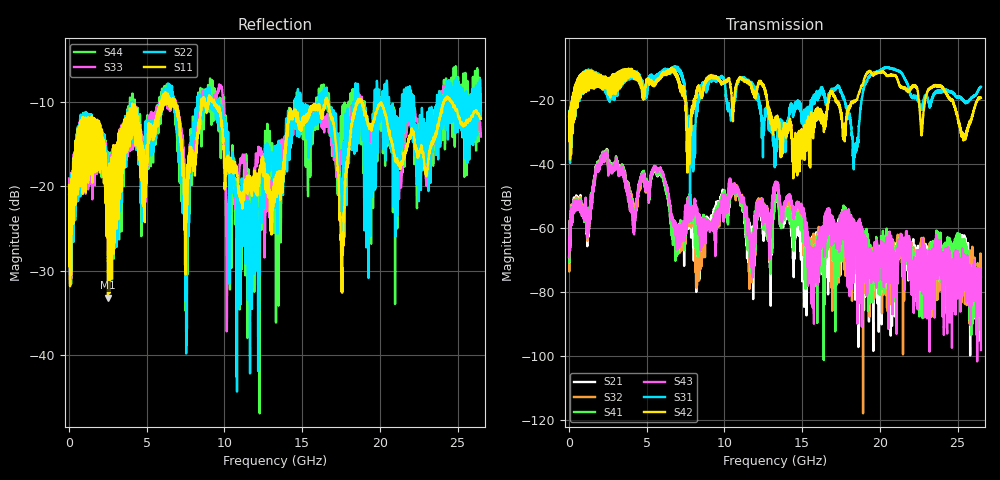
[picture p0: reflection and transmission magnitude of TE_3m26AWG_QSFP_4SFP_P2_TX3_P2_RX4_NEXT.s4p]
!Agilent Technologies,N5222A,MY51421691,A.10.00.00
!Agilent N5222A: A.10.00.00
!Date: Friday, January 30, 2015 12:36:14
!Correction: S11(Full 4 Port(1,2,3,4))
!S12(Full 4 Port(1,2,3,4))
!S13(Full 4 Port(1,2,3,4))
!S14(Full 4 Port(1,2,3,4))
!S21(Full 4 Port(1,2,3,4))
!S22(Full 4 Port(1,2,3,4))
!S23(Full 4 Port(1,2,3,4))
!S24(Full 4 Port(1,2,3,4))
!S31(Full 4 Port(1,2,3,4))
!S32(Full 4 Port(1,2,3,4))
!S33(Full 4 Port(1,2,3,4))
!S34(Full 4 Port(1,2,3,4))
!S41(Full 4 Port(1,2,3,4))
!S42(Full 4 Port(1,2,3,4))
!S43(Full 4 Port(1,2,3,4))
!S44(Full 4 Port(1,2,3,4))
!S4P File: Measurements: <S11,S12,S13,S14>,
!<S21,S22,S23,S24>,
!<S31,S32,S33,S34>,
!<S41,S42,S43,S44>:
# Hz S  dB  R 50.0
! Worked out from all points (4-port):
!   2650 points, 10 MHz to 26.5 GHz, reference 50 ohm
!   strongest paths, dB at 10 MHz, 6.63 GHz, 13.26 GHz, 19.88 GHz, 26.5 GHz:
!     S42: -24.9, -10.9, -25.3, -11.2, -19.2
!     S31: -24.9, -10.4, -34.3, -10.8, -15.7
!     S43: -69.1, -56.1, -45.6, -74.8, -98.1
!     S41: -68.6, -60.4, -49.7, -70.2, -75.3
!     S32: -63.8, -57.3, -46.4, -75.2, -75.3
!     S21: -69.2, -59.7, -50.3, -73.7, -72.5
!   lowest |S11| = -33.2 dB at 2.51 GHz (marker M1), VSWR 1.04, Z = 51 - j1.95 ohm
!   |S11| at or under -10 dB: start of sweep to 5.869 GHz; 9.354 GHz to 16.5 GHz (7.144 GHz wide, 55.3 % of centre); 20.09 GHz to 24.09 GHz (4.009 GHz wide, 18.1 % of centre)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
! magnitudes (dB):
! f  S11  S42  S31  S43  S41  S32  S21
! 10 MHz  -19.8  -24.9  -24.9  -69.1  -68.6  -63.8  -69.2
! 2.51 GHz  -33.2  -17.8  -19.7  -40.7  -39.6  -40.0  -39.3
! 8.28 GHz  -14.2  -16.4  -20.0  -55.5  -61.0  -68.2  -65.0
! 11.78 GHz  -20.8  -16.6  -14.4  -72.3  -68.0  -69.2  -69.8
! 13.34 GHz  -19.7  -25.1  -32.6  -45.7  -49.8  -46.2  -50.2
! 15.67 GHz  -10.8  -31.0  -19.2  -69.7  -68.8  -68.3  -62.5
! 26.5 GHz  -11.9  -19.2  -15.7  -98.1  -75.3  -75.3  -72.5
